(* Logix 5000 DataType export MPE_Output; software revision 33.01 *)

TYPE MPE_Output :   // MPE Output Data Type
STRUCT
   SetpointCurr : REAL;   // Set Current Setpoint
   SetpointVolt : REAL;   // Set Voltage Setpoint
END_STRUCT
END_TYPE
